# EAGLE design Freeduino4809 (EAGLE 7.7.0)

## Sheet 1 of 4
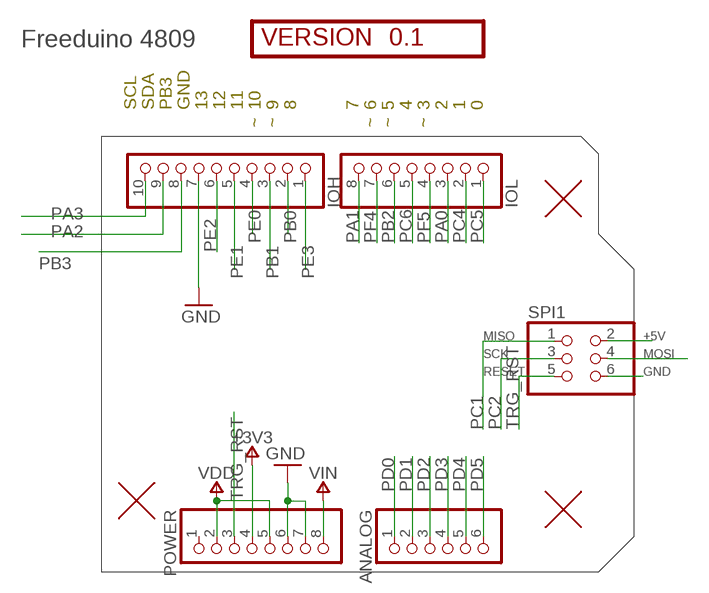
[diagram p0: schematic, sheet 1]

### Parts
ANALOG  Analog  PINHD-1X06TH  [1X06-TH]
IOH  Digital  PINHD-1X10TH  [1X10]
IOL  Digital  PINHD-1X08-DIGITALTH  [1X08]
POWER  Power  PINHD-1X08-POWERTH  [1X08]
SPI1  -  PINHD-2X03-ICSPTH  [2X03]
U$1  FIDUCIAL1.5X3  [FIDUCIAL-1.5X3]
U$2  FIDUCIAL1.5X3  [FIDUCIAL-1.5X3]
U$3  FIDUCIAL1.5X3  [FIDUCIAL-1.5X3]
VERSION  0.1  VERSION  [VERSION-NUMBER]

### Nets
+3V3: POWER.4 ; also sheet 4
GND: IOH.7 POWER.6 POWER.7 SPI1.6 ; also sheet 2,3,4
PA0: IOL.3 ; also sheet 2
PA1: IOL.8 ; also sheet 2
PA2: IOH.9 ; also sheet 2
PA3: IOH.10 ; also sheet 2
PB0: IOH.2 ; also sheet 2
PB1: IOH.3 ; also sheet 2
PB2: IOL.6 ; also sheet 2
PB3: IOH.8 ; also sheet 2
PC0: SPI1.4 ; also sheet 2
PC1: SPI1.1 ; also sheet 2
PC2: SPI1.3 ; also sheet 2
PC4: IOL.2 ; also sheet 2
PC5: IOL.1 ; also sheet 2
PC6: IOL.5 ; also sheet 2
PD0: ANALOG.1 ; also sheet 2
PD1: ANALOG.2 ; also sheet 2
PD2: ANALOG.3 ; also sheet 2
PD3: ANALOG.4 ; also sheet 2
PD4: ANALOG.5 ; also sheet 2
PD5: ANALOG.6 ; also sheet 2
PE0: IOH.4 ; also sheet 2
PE1: IOH.5 ; also sheet 2
PE2: IOH.6 ; also sheet 2
PE3: IOH.1 ; also sheet 2
PF4: IOL.7 ; also sheet 2
PF5: IOL.4 ; also sheet 2
TRG_RST: POWER.3 SPI1.5 ; also sheet 2,3
VDD [power]: POWER.2 POWER.5 SPI1.2 ; also sheet 2,3,4
VIN_EXT [power]: POWER.8 ; supply symbol labelled VIN ; also sheet 4
Unconnected: POWER.1

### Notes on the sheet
- Freeduino 4809
- SCL | SDA | PB3 | GND | 13 | 12 | 11 | 10 | 9 | 8 | 7 | 6 | 5 | 4 | 3 | 2 | 1 | 0
- ~ | ~ | ~ | ~ | ~

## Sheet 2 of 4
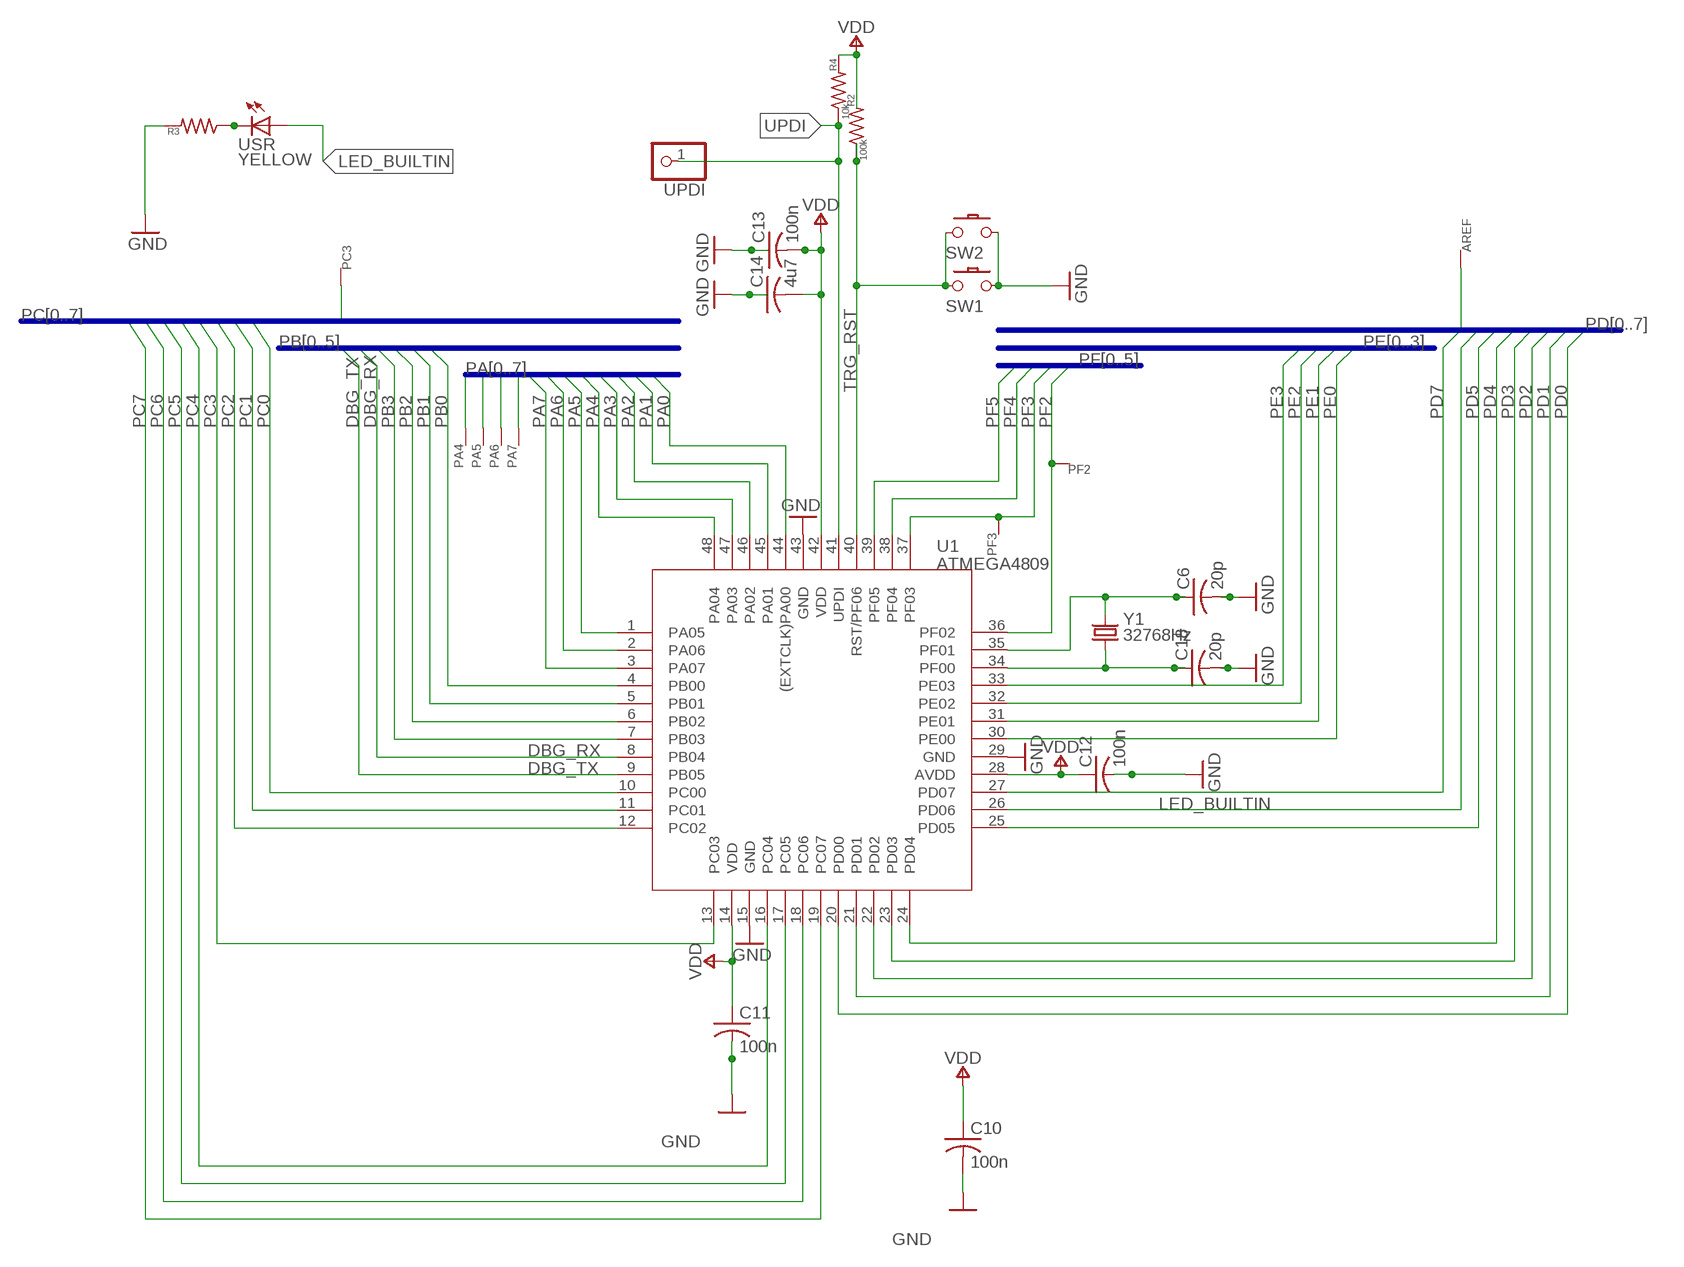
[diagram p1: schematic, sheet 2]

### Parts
AREF  WIRE-R10  [VIA10]
C6  20p  C-USC0805  [C0805]
C10  100n  C-USC0805  [C0805]
C11  100n  C-USC0805  [C0805]
C12  100n  C-USC0805  [C0805]
C13  100n  C-USC0805  [C0805]
C14  4u7  C-USC0805  [C0805]
C18  20p  C-USC0805  [C0805]
PA4  WIRE-R6  [VIA6]
PA5  WIRE-R6  [VIA6]
PA6  WIRE-R6  [VIA6]
PA7  WIRE-R6  [VIA6]
PC3  WIRE-R6  [VIA6]
PF2  WIRE-R6  [VIA6]
PF3  WIRE-R6  [VIA6]
R2  100k  R-US_R0805  [R0805]
R3  R-US_R0805  [R0805]
R4  10k  R-US_R0805  [R0805]
SW1  SW-PB2-NS/4MM  [SW-PB-SMT4MM]
SW2  SW-PB2-NSS52MM\  [SW-PB-SMT52MM]
U1  ATMEGA4809  [TQFP48]
UPDI  PINHD-1X1  [1X01]
USR  YELLOW  LED-YELLOW-0805  [CHIPLED_0805]
Y1  32768Hz  32.768KHZ  [ABS07]

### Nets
DBG_RX: U1.8(PB04) ; also sheet 3
DBG_TX: U1.9(PB05) ; also sheet 3
GND: C6.2 C10.2 C11.2 C12.2 C13.1 C14.1 C18.2 R3.2 SW1.P$4 SW2.S1 U1.15(GND) U1.29(GND) U1.43(GND) ; also sheet 1,3,4
LED_BUILTIN: U1.26(PD06) USR.A
N$4: C18.1 U1.34(PF00) Y1.1
N$5: C6.1 U1.35(PF01) Y1.2
N$22: R3.1 USR.C
PA0: U1.44((EXTCLK)PA00) ; also sheet 1
PA1: U1.45(PA01) ; also sheet 1
PA2: U1.46(PA02) ; also sheet 1
PA3: U1.47(PA03) ; also sheet 1
PA4: PA4.P$1 U1.48(PA04)
PA5: PA5.P$1 U1.1(PA05)
PA6: PA6.P$1 U1.2(PA06)
PA7: PA7.P$1 U1.3(PA07)
PB0: U1.4(PB00) ; also sheet 1
PB1: U1.5(PB01) ; also sheet 1
PB2: U1.6(PB02) ; also sheet 1
PB3: U1.7(PB03) ; also sheet 1
PC0: U1.10(PC00) ; also sheet 1
PC1: U1.11(PC01) ; also sheet 1
PC2: U1.12(PC02) ; also sheet 1
PC3: PC3.P$1 U1.13(PC03)
PC4: U1.16(PC04) ; also sheet 1
PC5: U1.17(PC05) ; also sheet 1
PC6: U1.18(PC06) ; also sheet 1
PC7: U1.19(PC07)
PD0: U1.20(PD00) ; also sheet 1
PD1: U1.21(PD01) ; also sheet 1
PD2: U1.22(PD02) ; also sheet 1
PD3: U1.23(PD03) ; also sheet 1
PD4: U1.24(PD04) ; also sheet 1
PD5: U1.25(PD05) ; also sheet 1
PD7: AREF.P$1 U1.27(PD07)
PE0: U1.30(PE00) ; also sheet 1
PE1: U1.31(PE01) ; also sheet 1
PE2: U1.32(PE02) ; also sheet 1
PE3: U1.33(PE03) ; also sheet 1
PF2: PF2.P$1 U1.36(PF02)
PF3: PF3.P$1 U1.37(PF03)
PF4: U1.38(PF04) ; also sheet 1
PF5: U1.39(PF05) ; also sheet 1
TRG_RST: R2.1 SW1.P$2 SW2.C2 U1.40(RST/PF06) ; also sheet 1,3
UPDI: R4.1 U1.41(UPDI) UPDI.1
VDD [power]: C10.1 C11.1 C12.1 C13.2 C14.2 R2.2 R4.2 U1.14(VDD) U1.28(AVDD) U1.42(VDD) ; also sheet 1,3,4

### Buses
PA[0..7]
PB[0..5]
PF[0..5]
PE[0..3]
PD[0..7]
PC[0..7]

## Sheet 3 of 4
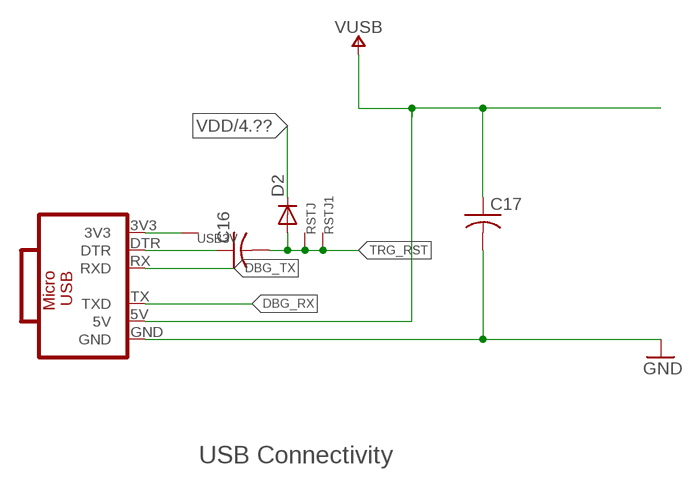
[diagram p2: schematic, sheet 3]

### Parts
C16  C-USC0805  [C0805]
C17  C-USC0805  [C0805]
D2  DIODE-SIGNAL-SOD323  [SOD323F]
RSTJ  WIRE-VIA8  [VIA8]
RSTJ1  WIRE-VIA8  [VIA8]
USB3V  WIRE-VIA8  [VIA8]
USBMOD  CH340E-MODNOHOLES  [CH340E-MOD-NOHOLES]

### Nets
DBG_RX: USBMOD.TX(TXD) ; also sheet 2
DBG_TX: USBMOD.RX(RXD) ; also sheet 2
DTR: C16.1 USBMOD.DTR
GND: C17.2 USBMOD.GND ; also sheet 1,2,4
TRG_RST: C16.2 D2.A RSTJ1.P$1 RSTJ.P$1 ; also sheet 1,2
USB3V: USB3V.P$1 USBMOD.3V3
VDD [power]: D2.C ; also sheet 1,2,4
VUSB: C17.1 USBMOD.5V ; also sheet 4

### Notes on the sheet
- USB Connectivity

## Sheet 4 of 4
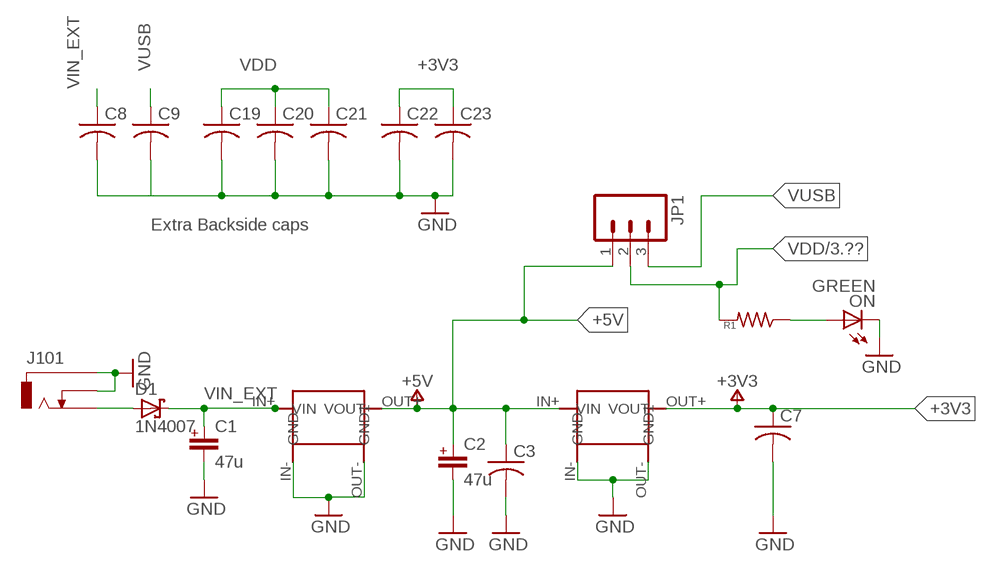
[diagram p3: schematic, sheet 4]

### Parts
C1  47u  C+-47UFPAN-D  [PANASONIC_D]
C2  47u  C+-47UFPAN-D  [PANASONIC_D]
C3  C-USC0805  [C0805]
C7  C-USC0805  [C0805]
C8  C-USC0805  [C0805]
C9  C-USC0805  [C0805]
C19  C-USC1206  [C1206]
C20  C-USC1206  [C1206]
C21  C-USC0805  [C0805]
C22  C-USC1206  [C1206]
C23  C-USC0805  [C0805]
D1  1N4007  D_SCHOTTKY-4007-SMB  [SMB_DO214AA]
J101  -  BARRELLG  [POWERSUPPLY_DC-21MM]
JP1  M03LOCK_LONGPADS  [1X03_LOCK_LONGPADS]
ON  GREEN  LED-GREEN-0805  [CHIPLED_0805]
R1  R-US_R0805  [R0805]
VREG-3V3  VREG-4-MOD  [VREG-4-11X17]
VREG-5V  VREG-4-MOD  [VREG-4-11X17]

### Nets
+3V3: C7.1 C22.1 C23.1 VREG-3V3.OUT+(VOUT) ; also sheet 1
+5V: C2.+ C3.1 JP1.1 VREG-3V3.IN+(VIN) VREG-5V.OUT+(VOUT)
GND: C1.- C2.- C3.2 C7.2 C8.2 C9.2 C19.2 C20.2 C21.2 C22.2 C23.2 J101.-1 J101.-2 J101.-3 J101.E1 J101.E2 J101.E3 ON.C VREG-3V3.IN-(GND) VREG-3V3.OUT-(GND1) VREG-5V.IN-(GND) VREG-5V.OUT-(GND1) ; also sheet 1,2,3
N$1: D1.A J101.+1 J101.+2 J101.+3
N$2: ON.A R1.1
VDD [power]: C19.1 C20.1 C21.1 JP1.2 R1.2 ; also sheet 1,2,3
VIN_EXT [power]: C1.+ C8.1 D1.C VREG-5V.IN+(VIN) ; also sheet 1
VUSB: C9.1 JP1.3 ; also sheet 3

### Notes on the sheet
- Extra Backside caps

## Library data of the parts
ANALOG = Arduino-connectors:PINHD-1X06: PIN HEADER; CODE-ARDUINO: 3649; DATASHEET: -; DISTRIBUTOR-LINK: -; DISTRIBUTOR-PN: -; MANUFACTURER: -; MANUFACTURER-PN: FH254-106DF085149V
AREF PA4-PA7 PC3 PF2 PF3 RSTJ RSTJ1 USB3V = mylib4:WIRE: Pad for a wire offboard
C1 C2 = Arduino-rcl:C+: Polarized Capacitor; CODE-ARDUINO: 0113; DATASHEET: https://industrial.panasonic.com/cdbs/www-data/pdf/RDE0000/DME0000COL90.pdf; DISTRIBUTOR-LINK: https://www.digikey.com/product-detail/en/panasonic-electronic-components/EEE-1EA470WP/PCE3908CT-ND/766284; DISTRIBUTOR-PN: PCE3908CT-ND; MANUFACTURER: Panasonic; MANUFACTURER-PN: EEE-1EA470WP; PN-ALTERNATIVE1: TS13C01E470MET000R
C3 C6-C14 C16-C23 = my-rcl:C-US: CAPACITOR, American symbol
D1 = Arduino-diodes:D_SCHOTTKY: Schottky Diodes; CODE-ARDUINO: 0020; DATASHEET: www.comchiptech.com/cms/UserFiles/CGRA4001-G%20Thru.%20CGRA4007-HF%20RevD.pdf; DISTRIBUTOR-LINK: https://www.digikey.com/product-detail/en/comchip-technology/CGRA4007-G/641-1018-1-ND/1121140; DISTRIBUTOR-PN: 641-1018-1-ND; MANUFACTURER: Comchip; MANUFACTURER-PN: CGRA4007-G; PN-ALTERNATIVE1: 1N4007SMA
D2 = mylib4:DIODE-SIGNAL
IOH = Arduino-connectors:PINHD-1X10: PIN HEADER; CODE-ARDUINO: 3648; DATASHEET: -; DISTRIBUTOR-LINK: -; DISTRIBUTOR-PN: -; MANUFACTURER: -; MANUFACTURER-PN: FH254-110DF085149V
IOL = Arduino-connectors:PINHD-1X08: PIN HEADER; CODE-ARDUINO: 3648; DATASHEET: -; DISTRIBUTOR-LINK: -; DISTRIBUTOR-PN: -; MANUFACTURER: -; MANUFACTURER-PN: FH254-108DF085149V
J101 = Arduino-connectors:BARREL: Power Barrel Connector Jack 2.10mm ID (0.083"), 5.50mm OD (0.217") Through Hole, Right Angle; CODE-ARDUINO: 0018; DATASHEET: http://www.mouser.com/ds/2/253/KC-301287-195995.pdf; DISTRIBUTOR-LINK: https://www.mouser.it/ProductDetail/Kobiconn/163-179PH-EX/?qs=Xb8IjHhkxj5l2UOaIqcGCw==; DISTRIBUTOR-PN: 163-179PH-EX; MANUFACTURER: Kobiconn; MANUFACTURER-PN: 163-179PH-EX
JP1 = SparkFun:M03: Header 3 Standard 3-pin 0.1" header. Use with straight break away headers (SKU : PRT-00116), right angle break away headers (PRT-00553), swiss pins (PRT-00743), machine pins (PRT-00117), and female headers (PRT-00115). Molex polarized connector foot print use with SKU : PRT-08232 with associated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
ON = Arduino-diodes:LED: LED; CODE-ARDUINO: 0043; DATASHEET: https://media.digikey.com/pdf/Data%20Sheets/Lite-On%20PDFs/LTST-C170GKT.pdf; DISTRIBUTOR-LINK: https://www.digikey.com/product-detail/it/lite-on-inc/LTST-C170GKT/160-1179-1-ND/269251; DISTRIBUTOR-PN: 160-1179-1-ND; MANUFACTURER: Lite-On; MANUFACTURER-PN: LTST-C170GKT; PN-ALTERNATIVE1: KPT-2012SGC
POWER = Arduino-connectors:PINHD-1X08: PIN HEADER; CODE-ARDUINO: 3649; DATASHEET: -; DISTRIBUTOR-LINK: -; DISTRIBUTOR-PN: -; MANUFACTURER: -; MANUFACTURER-PN: FH254-108DF085149V
R1-R4 = my-rcl:R-US_: RESISTOR, American symbol
SPI1 = Arduino-connectors:PINHD-2X03-ICSP: PIN HEADER; CODE-ARDUINO: 0114; DATASHEET: -; DISTRIBUTOR-LINK: https://www.digikey.com/product-detail/en/samtec-inc/TSW-103-25-S-D/TSW-103-25-S-D-ND/7863771; DISTRIBUTOR-PN: TSW-103-25-S-D-ND; MANUFACTURER: Samtec; MANUFACTURER-PN: TSW-103-25-S-D
SW1 SW2 = mylib4:SW-PB2-NS: SPST switch with no shield
U1 = Arduino-ucs&SoCs:ATMEGA4809: ATMEGA4809; CODE-ARDUINO: 2322; DATASHEET: http://ww1.microchip.com/downloads/en/DeviceDoc/40002016A.pdf; DISTRIBUTOR-LINK: https://www.digikey.com/product-detail/en/microchip-technology/ATMEGA4809-AFR/ATMEGA4809-AFRCT-ND/8540756; DISTRIBUTOR-PN: ATMEGA4809-AFRCT-ND; MANUFACTURER: Microchip; MANUFACTURER-PN: ATMEGA4809-AFR
U$1-U$3 = SparkFunEagle-6-6-07:FIDUCIAL: Fiducial Alignment Points
UPDI = pinhead:PINHD-1X1: PIN HEADER
USBMOD = mini-usb:CH340E-MOD
USR = Arduino-diodes:LED: LED; CODE-ARDUINO: 0044; DATASHEET: https://media.digikey.com/pdf/Data%20Sheets/Lite-On%20PDFs/LTST-C170GKT.pdf; DISTRIBUTOR-LINK: https://www.digikey.com/product-detail/it/lite-on-inc/LTST-C170YKT/160-1175-1-ND/269247; DISTRIBUTOR-PN: 160-1175-1-ND; MANUFACTURER: Lite-On; MANUFACTURER-PN: LTST-C170YKT; PN-ALTERNATIVE1: KPT-2012YC
VERSION = mylib4:VERSION: Version number for drawings
VREG-3V3 VREG-5V = mylib4:VREG-4-MOD
Y1 = Arduino-crystals:32.768KHZ: LF crystal; CODE-ARDUINO: 0213; DATASHEET: http://www.abracon.com/Resonators/ABS07.pdf; DISTRIBUTOR-LINK: http://www.digikey.com/product-detail/en/abracon-llc/ABS07-32.768KHZ-T/535-9542-1-ND/1237009; DISTRIBUTOR-PN: 535-9542-1-ND; MANUFACTURER: Abracon LLC; MANUFACTURER-PN: ABS07-32.768KHZ-T

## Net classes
0 default: width 0.2 mm, drill 0.5 mm
1 power: width 0.6 mm

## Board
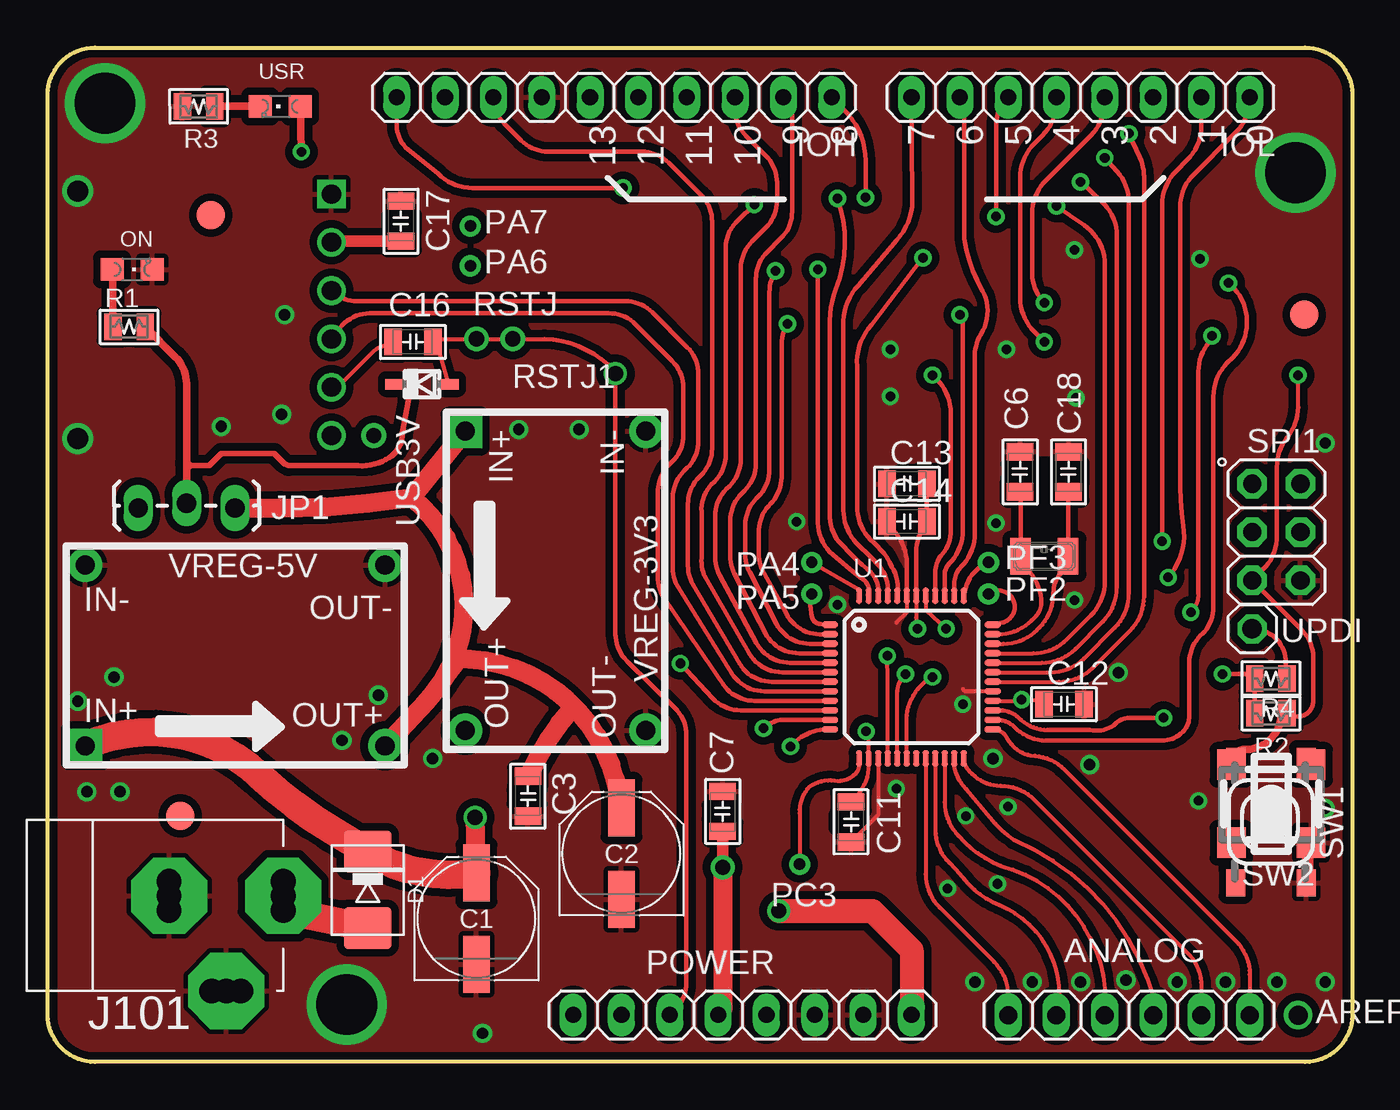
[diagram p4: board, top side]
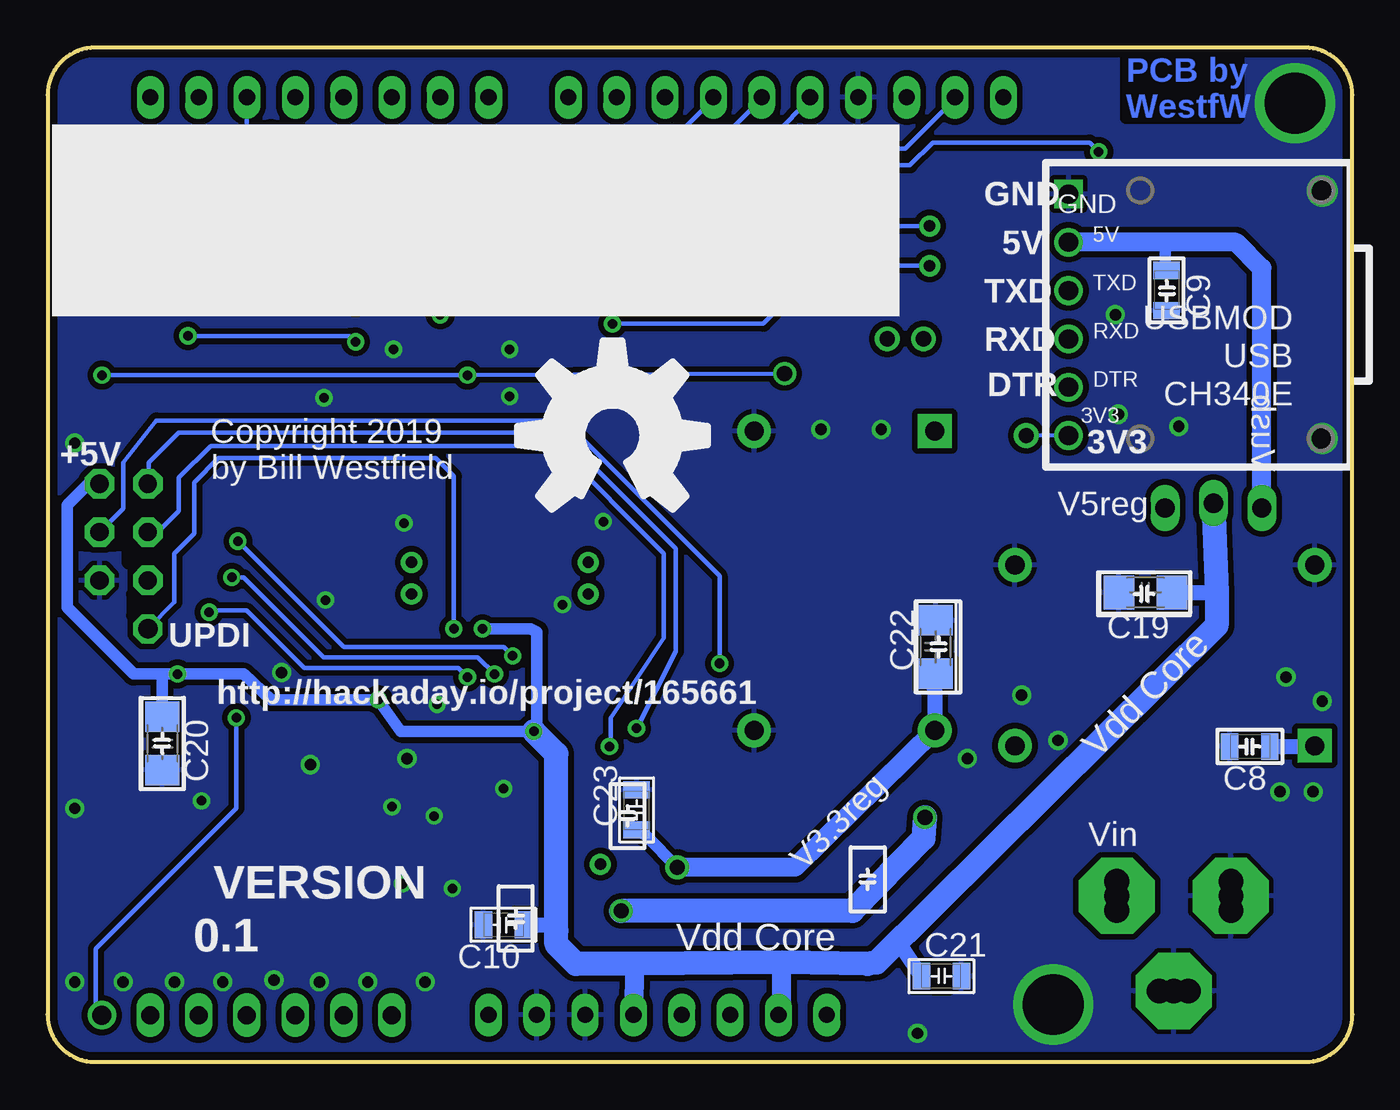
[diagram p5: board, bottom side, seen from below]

Size 68.58 x 53.34 mm. Coordinates in mm from the lower left corner, seen from the top.
Outline: 0,50.84 arc-90 2.5,53.34 66.08,53.34 arc-90 68.58,50.84 68.58,2.5 arc-90 66.08,0 2.5,0 arc-90 0,2.5 0,50.84
Copper layers (1*16): Top 0.035mm / dielectric 1.5mm / Bottom 0.035mm
Design rules "default *": minimum track width 8mil, minimum drill 0.3mm, track to track 6mil, track to pad 6mil, pad to pad 6mil, via to via 6mil, smd to smd 6mil, copper to edge 16mil, drill to drill 8mil, minimum pad ring 10mil, minimum via ring 8mil, stop-mask expansion 4mil, vias tented up to drill 0.55mm, thermal gap 10mil
tRestrict: area 52.1,25.6 to 52.8,30.5; area 50.5,30.7 to 51.8,31.4; area 53,30.8 to 54.4,31.5; area 51.8,30.7 to 53.1,31.4; area 44.8,29.7 to 45.5,31; area 44.8,27.8 to 45.6,29.1; area 18.8,37.2 to 19.5,38.6; area 17.9,43.8 to 19.3,44.5; area 34.8,12.8 to 36.1,13.5; area 41.4,12.3 to 42.8,13; area 24.5,13.6 to 25.9,14.3; area 3.9,38 to 4.6,39.3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
bRestrict: area 10.5,24 to 11.3,25.2; area 9,40.1 to 10.3,40.9; area 4.9,16 to 5.7,17.2; area 21.3,21.5 to 22.5,22.3; area 21.2,3.8 to 22,5.1; area 37.1,12.9 to 38.3,13.7; area 44.2,6.6 to 45,7.8; area 61.8,16.4 to 63.1,17.1; area 30.7,4.6 to 37.1,5.6; 6 lines

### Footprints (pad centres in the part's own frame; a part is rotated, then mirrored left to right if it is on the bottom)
1X06-TH = drill 0.95 pad 1.422 long: 1 -6.35,0; 2 -3.81,0; 3 -1.27,0; 4 1.27,0; 5 3.81,0; 6 6.35,0
VIA10 = drill 1: P$1 0,0
PANASONIC_D = smd 3 x 1.4: + 2.4,0; - -2.4,0
C0805 = smd 0.914 x 1.397: 1 -1.053,0; 2 1.053,0
C1206 = smd 1.6 x 1.8: 1 -1.4,0; 2 1.4,0
SMB_DO214AA = smd 2.2 x 2.5: A -2,0; C 2,0
SOD323F = smd 0.55 x 1.05: A 0,-1.4; C 0,1.4
1X10 = drill 0.85 pad 1.422 long: 1 -11.43,0; 2 -8.89,0; 3 -6.35,0; 4 -3.81,0; 5 -1.27,0; 6 1.27,0; 7 3.81,0; 8 6.35,0; 9 8.89,0; 10 11.43,0
1X08 = drill 0.85 pad 1.422 long: 1 -8.89,0; 2 -6.35,0; 3 -3.81,0; 4 -1.27,0; 5 1.27,0; 6 3.81,0; 7 6.35,0; 8 8.89,0
POWERSUPPLY_DC-21MM = drill 1.3 pad 4 octagon: +1 -0.076,-6.35; -1 -0.076,-0.356; E1 -5.08,-3.353 | drill 1.3: +2 -0.838,-6.35; +3 0.686,-6.35; -2 -0.838,-0.356; -3 0.686,-0.356; E2 -5.08,-2.591; E3 -5.08,-4.115
1X03_LOCK_LONGPADS = drill 1.016 long: 1 0,0; 2 2.54,-0.254; 3 5.08,0
CHIPLED_0805 = smd 1.2 x 1.2: A -1.05,0; C 1.05,0
VIA6 = drill 0.6: P$1 0,0
R0805 = smd 0.914 x 1.397: 1 -0.85,0; 2 0.85,0
VIA8 = drill 0.8: P$1 0,0
2X03 = drill 0.95 pad 1.55 octagon: 1 2.54,1.27; 2 2.54,-1.27; 3 0,1.27; 4 0,-1.27; 5 -2.54,1.27; 6 -2.54,-1.27
SW-PB-SMT4MM = smd 1.4 x 1: P$1 -3.2,1.85; P$2 -3.2,-1.85; P$3 3.2,-1.85; P$4 3.2,1.85
SW-PB-SMT52MM = smd 1.5 x 1.6: C1 2.1,2.05; C2 2.1,-2.05; S1 -2.1,2.05; S2 -2.1,-2.05
TQFP48 = smd 0.85 x 0.32: 1 -4.275,2.75; 2 -4.275,2.25; 3 -4.275,1.75; 4 -4.275,1.25; 5 -4.275,0.75; 6 -4.275,0.25; 7 -4.275,-0.25; 8 -4.275,-0.75; 9 -4.275,-1.25; 10 -4.275,-1.75; 11 -4.275,-2.25; 12 -4.275,-2.75; 25 4.275,-2.75; 26 4.275,-2.25; 27 4.275,-1.75; 28 4.275,-1.25; 29 4.275,-0.75; 30 4.275,-0.25; 31 4.275,0.25; 32 4.275,0.75; 33 4.275,1.25; 34 4.275,1.75; 35 4.275,2.25; 36 4.275,2.75 | smd 0.32 x 0.85: 13 -2.75,-4.275; 14 -2.25,-4.275; 15 -1.75,-4.275; 16 -1.25,-4.275; 17 -0.75,-4.275; 18 -0.25,-4.275; 19 0.25,-4.275; 20 0.75,-4.275; 21 1.25,-4.275; 22 1.75,-4.275; 23 2.25,-4.275; 24 2.75,-4.275; 37 2.75,4.275; 38 2.25,4.275; 39 1.75,4.275; 40 1.25,4.275; 41 0.75,4.275; 42 0.25,4.275; 43 -0.25,4.275; 44 -0.75,4.275; 45 -1.25,4.275; 46 -1.75,4.275; 47 -2.25,4.275; 48 -2.75,4.275 | smd 0 x 0: EP 0,0
FIDUCIAL-1.5X3 = smd 1.5 x 1.5: 1 0,0
1X01 = drill 1.016 octagon: 1 0,0
CH340E-MOD-NOHOLES = drill 1: 3V3 6.35,6.35; 5V 6.35,-3.81; DTR 6.35,3.81; RX 6.35,1.27; TX 6.35,-1.27 | drill 1 square: GND 6.35,-6.35
VREG-4-11X17 = drill 1 pad 1.778 square: IN+ -5,-2.5 | drill 1 pad 1.778: IN- -5,7; OUT+ 10.75,-2.5; OUT- 10.75,7
ABS07 = smd 1.1 x 1.9: 1 -1.25,0; 2 1.25,0

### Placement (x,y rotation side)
ANALOG  56.83,2.46 0 top
AREF  65.72,2.46 0 top
C1  22.54,7.54 90 top
C2  30.16,10.95 90 top
C3  25.24,13.97 270 top
C6  51.12,31.04 90 top
C7  35.48,13.18 90 top
C8  5.4,16.59 180 bottom
C9  9.76,40.56 270 bottom
C10  44.63,7.21 180 bottom
C11  42.23,12.62 270 top
C12  53.42,18.81 0 top
C13  45.16,30.4 0 top
C14  45.16,28.42 0 top
C16  19.21,37.86 0 top
C17  18.57,44.21 90 top
C18  53.66,31.04 90 top
C19  10.87,24.69 180 bottom
C20  62.55,16.75 270 bottom
C21  21.6,4.52 0 bottom
C22  21.91,21.83 90 bottom
C23  37.62,13.26 90 bottom
D1  16.83,9.05 90 top
D2  19.69,35.64 90 top
IOH  29.78,50.72 180 top
IOL  54.29,50.72 180 top
J101  6.03,8.81 90 top
JP1  9.84,29.13 180 top
ON  4.45,41.67 0 top
PA4  40.16,26.27 0 top
PA5  40.16,24.61 0 top
PA6  22.23,41.86 0 top
PA7  22.23,43.96 0 top
PC3  39.53,10.4 0 top
PF2  49.45,24.61 0 top
PF3  49.45,26.27 0 top
POWER  36.51,2.47 0 top
R1  4.29,38.66 0 top
R2  64.29,18.34 180 top
R3  7.94,50.24 180 top
R4  64.29,20.16 180 top
RSTJ  22.54,38.02 0 top
RSTJ1  24.45,38.02 0 top
SPI1  64.58,27.86 90 top
SW1  64.29,12.62 270 top
SW2  64.31,13.58 180 top
U1  45.4,20.24 0 top
U$1  6.99,12.94 0 top
U$2  66.04,39.29 0 top
U$3  8.57,44.53 0 top
UPDI  63.31,22.78 0 top
USB3V  17.14,32.94 0 top
USBMOD  8.57,39.29 180 bottom
USR  12.22,50.24 180 top
VERSION  not placed on the board
VREG-3V3  24.45,28.18 270 top
VREG-5V  6.99,19.13 0 top
Y1  52.39,26.59 180 top

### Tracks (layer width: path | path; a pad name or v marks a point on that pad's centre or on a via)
+3V3  (via drill 0.8 pad 1.27)
  Top 0.6: C7.1 v35.48,10.24
  Top 1: v35.48,10.24 35.48,2.71 POWER.4
  Bottom 0.6: C22.1 arc-90 21.95,19.46 | C23.1 37.13,11.88 v35.48,10.24
  Bottom 0.8: 21.95,19.46 VREG-3V3.OUT+
  Bottom 1: VREG-3V3.OUT+ 29.29,10.24 v35.48,10.24
+5V
  Top 0.6: 29.85,14.84 28.34,17.86 27.54,18.57 | 30.24,13.33 C2.+
  Top 1: C2.+ 30.24,13.35 | JP1.1 12.22,29.13 arc9 19.13,29.69 | VREG-5V.OUT+ 19.92,18.97 | 19.92,18.97 arc95 19.13,29.69 | 19.13,29.69 VREG-3V3.IN+ | 30.24,13.33 29.85,14.84 arc77 21.35,21.19 21.35,20.88 19.92,18.97 | C3.1 25.4,15.24 arc-17 27.54,18.57
DBG_RX
  Top 0.229: U1.8 37.66,19.49 arc-58 35.96,20.43 33.16,24.91 arc-32 32.86,25.97 32.86,29.65 arc-45 33.45,31.07 33.62,31.24 arc45 34.21,32.66 34.21,36.16 arc45 33.62,37.57 31.78,39.42 arc45 30.37,40 16.26,40 arc-45 USBMOD.TX
DBG_TX
  Top 0.229: U1.9 37.15,18.99 arc-56 35.5,19.86 32.5,24.25 arc-34 32.07,25.38 32.07,30.05 arc-45 32.73,31.46 32.83,31.56 arc45 33.42,32.98 33.42,35.45 arc45 32.83,36.86 30.91,38.78 arc45 29.49,39.37 16.94,39.37 arc53 15.35,38.58 USBMOD.RX
DTR
  Top 0.203: USBMOD.DTR 15.24,35.48 17.08,37.33 arc-45 18,37.7 C16.1
GND  (via drill 0.5, 0.6, 1.1, 3.2)
  Top 0.203: U1.15 43.65,12.99 C11.2 | U1.29 48.22,19.49 48.1,19.61 | U1.43 45.15,23.64 44.61,23.1
  Top 0.229: U1.43 45.15,26.24 arc45 44.45,27.94 arc45 44.35,28.17 C14.1
  Top 0.6: SW2.S1 arc90 66.22,11.33 66.22,9.29
  other vias: 54.29,4.21 56.68,4.31 59.37,4.21 61.91,4.21 47.31,9.13 49.69,15.95 50.48,13.41 48.26,12.94 51.75,4.21 49.93,9.37 54.77,15.64 56.28,20.48 64.61,4.21 48.74,4.21 41.51,24.05 48.1,18.81 44.61,14.37 44.29,37.47 44.29,35 54.05,34.93 50.4,37.47 53.97,42.7 60.56,42.23 39.37,28.42 49.85,28.34 53.97,24.29 1.59,45.8 1.59,32.78 67.15,4.21 67.15,13.34 67.15,32.54 1.59,18.97 3.49,20.24 3.81,14.21 2.06,14.21 22.86,1.51 24.77,33.26 27.94,33.26 20.24,15.95 60.48,13.73 9.13,33.42 12.3,34.05 12.46,39.29 17.38,19.29 15.48,16.91 3.02,50.42 65.58,46.77 15.72,3.02
  pour Top (isolate 0.4): -2.86,55.8 72.71,55.8 72.71,-3.25 -2.86,-3.25
  pour Bottom (isolate 0.3): -0.64,55.17 70.17,55.17 70.17,-1.98 -0.64,-1.98 -0.64,53.26
LED_BUILTIN  (via drill 0.5)
  Top 0.203: U1.26 49.93,17.99 arc-45 50.78,17.64 arc45 52.47,16.91
  Top 0.229: v62.07,40.96 62.21,40.83 arc-47 63.02,38.98 63.02,38.82 arc-45 62.29,37.05 62.01,36.77 arc45 61.28,35 61.28,23.93 arc-45 60.69,22.51 60.59,22.41 arc45 60.01,21 60.01,18.19 arc-45 59.66,17.36 arc-45 58.58,16.91 52.47,16.91
  Top 0.4: USR.A v13.33,47.86
  Bottom 0.229: v62.07,40.96 62.07,41.04 54.93,41.04 54.45,41.51 47.7,41.51 46.67,40.48 42.78,40.48 40,43.74 34.45,43.74 31.09,47.09 arc45 30.96,47.15 23.26,47.15 22.07,48.34 13.81,48.34 v13.33,47.86
N$1
  Top 1.5: J101.+2 D1.A
  Bottom 0.2: J101.+2 J101.+1 | J101.+3 J101.+1 | 12.38,7.94 J101.+1
N$2
  Top 0.4: ON.A 3.44,40.84 R1.1
N$4
  Top 0.203: U1.34 50.24,21.99 arc45 52.01,22.72 52.13,22.84 arc45 52.86,24.61 52.86,24.65
  Top 0.229: C18.1 53.64,29.96 Y1.1 53.34,26.29 53.34,25.8 arc45 52.86,24.65
N$5
  Top 0.203: U1.35 49.95,22.49 arc45 51.72,23.22 51.95,23.45 arc45 52.23,24.13
  Top 0.229: C6.1 51.14,29.96 Y1.2 51.43,26.29 51.43,25.96 51.5,25.89 arc-45 52.23,24.13
N$22
  Top 0.4: R3.1 USR.C
PA0  (via drill 0.5)
  Top 0.229: v46.01,42.28 43.31,38.78 arc46 42.54,36.58 42.54,29.23 arc49 43.42,27.3 arc-26 44.37,26.03 arc-40 U1.44
  Bottom 0.229: IOL.3 58.1,48.34 53.18,43.42 46.99,43.42 v46.01,42.28
PA1
  Top 0.229: IOL.8 45.45,45.54 arc-46 44.63,43.22 42.6,40.83 arc46 41.83,38.72 41.83,29.01 arc43 42.51,27.3 42.74,27.05 arc-2 43.64,26.17 arc-49 U1.45
PA2  (via drill 0.5)
  Top 0.229: U1.46 arc62 43.06,25.94 arc-7 42.34,26.57 41.57,27.37 arc-44 41.12,29.02 41.12,38.97 arc-22 41.43,40.64 arc41 v41.51,45.4
  Bottom 0.229: 41.47,45.44 v41.51,45.4 40.56,46.35 33.26,46.35 31.59,48.02 23.49,48.02 20.96,50.56 20.96,50.72 IOH.9
PA3  (via drill 0.5)
  Top 0.203: U1.47 arc-90 43.1,24.57 43.18,24.84
  Top 0.229: v40.48,41.67 40.48,28.55 arc44 41.1,26.82 arc2 42.7,25.48 arc-53 43.18,24.84 | v30.24,45.96 22.32,45.96 arc-45 20.53,46.7 18.81,48.1 arc-45 18.35,49.38 IOH.10
  Bottom 0.229: v40.48,41.67 40.32,41.91 39.45,42.78 33.42,42.78 v30.24,45.96
PA4
  Top 0.203: U1.48 42.62,24.84
  Top 0.229: 42.62,24.84 PA4.P$1
PA5
  Top 0.229: U1.1 40.64,23.02 arc-73 40.16,23.42 arc-27 PA5.P$1
PA6  (via drill 0.5)
  Top 0.229: U1.2 40.6,22.49 arc-63 38.81,23.58 38.66,23.89 37.54,25.91 arc-28 37.39,26.93 37.39,27.83 arc-45 37.89,29.24 37.99,29.34 arc45 38.58,30.75 38.58,37.73 arc-30 38.84,38.72 v38.89,38.81
  Bottom 0.229: v38.89,38.81 30.96,38.81 27.91,41.86 PA6.P$1
PA7  (via drill 0.5)
  Top 0.229: U1.3 40.07,21.99 arc-63 38.29,23.07 36.9,25.76 arc-27 36.67,26.68 36.67,28.22 arc-45 37.26,29.64 37.36,29.74 arc45 37.94,31.15 37.94,40.49 arc-27 38.15,41.38 v38.26,41.59
  Bottom 0.229: v38.26,41.59 30.8,41.59 28.43,43.96 PA7.P$1
PB0
  Top 0.229: U1.4 39.49,21.49 arc-63 37.72,22.57 36.1,25.68 arc-27 35.88,26.6 35.88,28.46 arc-45 36.46,29.88 36.64,30.05 arc45 37.23,31.47 37.23,41.16 arc-45 37.81,42.58 38.55,43.31 arc45 39.13,44.72 39.13,49.61 arc45 IOH.2
PB1
  Top 0.229: U1.5 39.02,20.99 arc-61 37.26,22.04 35.33,25.59 arc-29 35.08,26.54 35.08,28.7 arc-45 35.67,30.11 35.85,30.29 arc45 36.43,31.71 36.43,41.72 arc-45 37.02,43.13 37.75,43.86 arc45 38.34,45.28 38.34,46.24 arc45 37.75,47.66 36.7,48.71 arc-45 36.12,50.12 36.12,50.7 IOH.3
PB2  (via drill 0.5)
  Top 0.229: v49.85,44.45 49.85,49.19 arc-45 IOL.6 | U1.6 38.61,20.49 arc-60 36.88,21.49 34.56,25.49 arc-30 34.37,26.49 34.37,28.94 arc-45 34.88,30.35 35.05,30.53 arc45 35.64,31.94 35.64,42.8 arc-47 36.26,44.25 v37.15,45.08
  Bottom 0.229: v37.15,45.08 40,45.08 40.96,44.13 45.4,44.13 45.72,44.45 v49.85,44.45
PB3
  Top 0.229: U1.7 38.07,19.99 arc-60 36.34,20.98 33.93,25.09 arc-30 33.65,26.1 33.65,29.33 arc-45 34.24,30.75 34.34,30.85 arc45 34.92,32.26 34.92,44.18 arc45 34.34,45.59 32.65,47.28 arc45 31.24,47.86 26.31,47.86 arc-45 24.89,48.45 24,49.34 arc-45 IOH.8
PC0  (via drill 0.5)
  Top 0.229: U1.10 36.43,18.49 arc-47 34.97,19.12 v33.26,20.95
  Bottom 0.229: v33.26,20.95 33.26,25.56 41.43,33.73 62.86,33.73 64.61,31.51 64.61,29.1 SPI1.4
PC1  (via drill 0.5)
  Top 0.229: v37.62,17.54 arc-29 38.28,17.93 arc-16 38.71,17.99 U1.11
  Bottom 0.229: SPI1.1 63.26,30.45 63.26,31.51 61.67,33.1 41.67,33.1 35.56,26.99 35.56,21.59 v37.62,17.54
PC2  (via drill 0.5)
  Top 0.203: 40.99,17.49 U1.12
  Top 0.229: v39.05,16.59 39.22,16.76 arc-20 39.91,17.25 | 39.91,17.25 arc-25 40.99,17.49 | 39.93,17.22 39.91,17.25
  Bottom 0.229: 62.86,27.86 SPI1.3 62.79,27.86 61.67,28.97 61.67,30.72 60.01,32.38 41.83,32.38 36.2,26.75 36.2,22.3 38.97,18.1 38.97,16.67 v39.05,16.59
PC3
  Top 0.203: U1.13 42.65,15.65 arc-45 42.44,15.13 arc-45 41.55,14.76 arc45 40.02,14.46 arc45 39.53,13.09 PC3.P$1
PC4  (via drill 0.5)
  Top 0.203: U1.16 44.15,20.06 v44.13,21.35
  Top 0.229: IOL.2 60.64,49.22 arc-45 59.91,47.45 59.31,46.85 arc45 58.58,45.08 v58.58,27.38
  Bottom 0.229: v44.13,21.35 44.61,21.83 53.02,21.83 v58.58,27.38
PC5  (via drill 0.5)
  Top 0.203: U1.17 44.65,19.36 arc-45 v45.09,20.4
  Top 0.229: IOL.1 63.18,50.64 arc-45 62.45,48.88 60.1,46.53 arc45 59.53,44.68 59.53,30.24 arc9 59.69,28.18 arc-50 v58.9,25.48
  Bottom 0.229: v45.09,20.4 45.96,21.27 54.05,21.27 58.26,25.48 v58.9,25.48
PC6  (via drill 0.5)
  Top 0.203: 60.48,24.61 arc-45 v60.09,23.65 | U1.18 45.15,18 arc-45 45.88,19.77 46.35,20.24 v46.51,20.24
  Top 0.229: 60.48,24.61 60.48,36.3 arc-45 61.2,38.02 v61.2,38.18 | v52.39,37.86 51.85,38.4 arc-45 51.12,40.17 51.12,46.51 arc-45 51.85,48.28 52.29,48.72 arc45 53.02,50.49 IOL.5
  Bottom 0.229: v61.2,38.18 52.71,38.18 v52.39,37.86 | v46.51,20.24 46.99,20.72 55.09,20.72 58.1,23.73 60.01,23.73 v60.09,23.65
PD0
  Top 0.203: U1.20 46.15,9.89 arc45 46.88,8.12 49.75,5.26 arc-45 50.48,3.49 ANALOG.1
PD1
  Top 0.203: U1.21 46.67,15.95 46.67,12.23 arc45 47.4,10.46 arc-6 48.18,9.6 arc28 50.01,8.25 arc-54 53.02,4.76 arc-28 ANALOG.2
PD2
  Top 0.203: U1.22 47.15,13.65 arc45 47.88,11.88 arc27 50.09,10.32 arc-81 ANALOG.3
PD3
  Top 0.203: ANALOG.4 58.15,3.27 arc52 50.8,11.67 arc-17 49.53,12.86 48.29,14.34 arc-45 47.63,15.94 U1.23
PD4
  Top 0.203: U1.24 arc45 48.42,15.32 48.6,15.14 arc45 50.08,14.53 arc-45 51.85,13.79 59.91,5.73 arc-45 60.64,3.96 ANALOG.5
PD5
  Top 0.203: U1.25 arc-58 50.38,17.1 50.55,16.83 arc45 51.67,16.11 arc-45 53.44,15.38 62.45,6.37 arc-45 63.18,4.6 ANALOG.6
PD7  (via drill 0.5)
  Top 0.203: U1.27 50.07,18.49 arc-45 51.02,18.12 arc45 52.55,17.46
  Top 0.229: 52.55,17.46 54.79,17.46 arc45 56.04,17.7 arc-45 56.84,18.1 v58.66,18.1
  Bottom 0.229: v58.66,18.1 58.66,13.33 66.04,5.95 66.04,2.78 AREF.P$1 65.56,2.46
PE0  (via drill 0.5)
  Top 0.203: U1.30 53.17,19.99 arc45 54.93,20.72 56.89,22.68 arc45 57.63,24.45
  Top 0.229: 57.63,24.45 57.63,46.53 arc24 57.4,47.56 v56.83,48.82
  Bottom 0.229: IOH.4 33.65,50.72 33.65,50.56 35.72,48.5 54.05,48.5 54.37,48.82 v56.83,48.82
PE1  (via drill 0.5)
  Top 0.203: U1.31 52.71,20.49 arc45 54.48,21.22 56.1,22.84 arc45 56.83,24.61
  Top 0.229: 56.83,24.61 56.83,45.17 arc42 56.2,46.83 v55.56,47.55
  Bottom 0.229: v55.56,47.55 44.48,47.55 44.25,47.78 33.89,47.78 31.12,50.56 31.12,50.72 IOH.5
PE2  (via drill 0.5)
  Top 0.203: U1.32 52.26,20.99 arc45 54.03,21.72 55.47,23.16 arc45 56.2,24.93
  Top 0.229: 56.2,24.93 56.2,43.43 arc47 55.39,45.27 v54.29,46.28
  Bottom 0.229: 28.57,50.72 IOH.6 28.5,50.64 30.4,48.74 31.91,48.74 33.58,47.07 43.84,47.07 44.16,46.75 53.82,46.75 v54.29,46.28
PE3  (via drill 0.5)
  Top 0.203: U1.33 51.81,21.49 arc45 53.58,22.22 54.83,23.48
  Top 0.229: 54.83,23.48 arc45 55.56,25.24 55.56,41.94 arc55 54.48,44 v53.02,45.01 | v42.99,45.45 42.99,47.4 arc45 41.88,50.06 IOH.1
  Bottom 0.229: v53.02,45.01 51.91,45.88 43.51,45.88 v42.99,45.45
PF2
  Top 0.229: U1.36 50.17,23.1 arc206 PF2.P$1
PF3
  Top 0.229: U1.37 48.26,24.92 arc-53 PF3.P$1
PF4
  Top 0.229: U1.38 47.65,25.17 arc-45 48,26.02 arc45 48.74,27.78 48.74,37.15 arc-32 49.05,38.26 arc60 49.13,40.56 arc-22 48.18,43.28 48.18,50.64 IOL.7
PF5  (via drill 0.5)
  Top 0.229: U1.39 47.15,25.65 arc-45 47.37,26.18 arc45 48.1,27.94 48.1,39.13 v47.94,39.29 | v52.39,39.93 arc-45 51.75,41.46 51.75,44.6 arc-45 52.48,46.37 54.83,48.72 arc45 55.56,50.49 IOL.4
  Bottom 0.229: v47.94,39.29 48.58,39.93 v52.39,39.93
TRG_RST  (via drill 0.5, 0.8)
  Top 0.203: 65.72,34.43 v65.72,36.12 | 32.62,2.55 POWER.3 | D2.A 20.45,37.86 C16.2 20.26,38.02 RSTJ.P$1 RSTJ1.P$1 26.11,38.02
  Top 0.229: 65.72,34.43 arc-38 65.2,32.9 65.14,32.82 arc38 64.61,31.29 64.61,27.66 arc-45 63.88,25.89 SPI1.5 65.93,22.7 arc-45 66.52,21.29 66.52,18.97 arc-90 65.72,18.18 65.3,18.18 arc-90 R2.1 64.83,18.23 | 26.11,38.02 arc-45 29.78,36.34 v29.85,36.19 29.85,22.51 arc46 30.45,21.08 32.97,18.61 arc-46 33.58,17.18 33.58,4.18 arc-45 32.99,2.76 POWER.3 | U1.40 46.65,25.74 arc-45 47.05,26.73 arc45 47.47,28.1 47.47,34.13 arc45 46.73,35.9 v46.51,36.12 | SW1.P$2 62.36,15.82
  Top 0.4: 62.36,15.82 arc-90 62.86,16.43 arc90 64.83,18.23
  Top 0.6: SW2.C2 SW1.P$2
  Bottom 0.229: v65.72,36.12 v46.51,36.12 v29.85,36.19
UPDI  (via drill 0.5)
  Top 0.203: U1.41 46.15,23.78 v47.23,22.78
  Top 0.229: R4.1 arc-90 65.09,20.22 65.09,21 arc90 UPDI.1
  Bottom 0.203: 61.91,24.18 UPDI.1
  Bottom 0.229: 61.91,24.18 61.91,26.75 60.88,27.78 60.88,30.48 59.61,31.75 48.18,31.75 47.23,30.8 v47.23,22.78
USB3V
  Bottom 0.203: USBMOD.3V3 USB3V.P$1
VDD  (via drill 0.5)
  Top 0.203: C11.1 42.42,13.87 arc45 43.15,15.63 U1.14 43.15,17.2 v43.02,17.38 | U1.42 45.65,23.35 v45.72,22.78 | D2.C 18.64,35.61 arc-45 18.97,34.87 | U1.28 50.78,18.99 v51.2,19.05 52.13,19.05 C12.1 52.29,18.57
  Top 0.229: C13.2 C14.2 46.05,28.15 arc33 45.65,26.8 U1.42 | R2.2 R4.2 arc45 62.87,20.4 v61.75,20.4
  Top 0.3: 18.97,34.87 18.65,33.06 arc-53 17.97,31.77 arc-37 16.31,31.35 12.67,31.35 12.47,31.44 12.15,31.76 | 12.15,31.76 | 12.15,31.76 11.91,32 9.13,32 8.49,31.35 7.46,31.35
  Top 0.4: R1.2 6.72,37.08 arc-45 7.3,35.66 7.3,31.51 | 7.3,31.51 JP1.2 | 7.46,31.35 arc-90 7.3,31.51
  Bottom 0.6: v45.72,22.78 43.18,22.78 42.86,22.62 42.86,17.86 43.02,17.7 v43.02,17.38 50.01,17.38 v51.2,19.05 56.83,19.05 58.26,20.4 v61.75,20.4 62.55,20.4 | 62.55,20.4 64.06,20.4 67.55,23.89 67.55,29.29 66.44,30.4 SPI1.2 | C20.1 62.55,20.4
  Bottom 0.8: C19.1 7.14,24.69 | C21.1 23.81,6.25 25.48,5.16 | C10.1 42.15,7.21 41.84,6.91
  Bottom 1: POWER.2 30,2.47 30,5.24 | POWER.5 37.7,5.16
  Bottom 1.27: JP1.2 7.14,24.69 | 7.14,24.69 7.14,22.94 25,5.24 25.48,5.16 30,5.24 37.7,5.16 40.81,5.16 41.84,6.19 41.84,6.91 41.84,16.21 v43.02,17.38 | 7.14,24.69 arc-90 7.14,24.69
VIN_EXT  (via drill 0.8)
  Top 1: C1.+ arc90 C1.+ v22.47,12.86
  Top 1.27: v38.43,7.94 43.35,7.94 45.42,5.88 45.42,2.49 POWER.8
  Top 1.5: VREG-5V.IN+ arc-67 11.11,15.08 arc12 15,12.14 D1.C arc40 C1.+
  Bottom 0.6: 2.02,16.59 arc-90 VREG-5V.IN+
  Bottom 0.8: C8.1 2.02,16.59
  Bottom 1.27: v22.47,12.86 22.55,11.75 26.28,7.94 v38.43,7.94
VUSB
  Top 0.6: C17.1 14.98,43.16 USBMOD.5V
  Bottom 0.6: C9.1 arc90 9.84,41.69 9.84,43.1
  Bottom 1: JP1.3 4.76,41.75 6.11,43.1 9.84,43.1 USBMOD.5V

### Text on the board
Bottom: PCB by / WestfW
tPlace: 13 | 12 | 11 | 10 | 9 | 8 | 7 | 6 | 5 | 4 | 3 | 2 | 1 | 0
History: 20190605 by WestfW: Tag at "Version 0.1" | 20190603 by WestfW: dual footprints for reset switch. Connect Vin. | 20190602 by WestfW: Add fiducuals. Tweak silkscreen, backside cap packages. | 20190523 by WestfW: remove Aref, add backside bypass caps, simplify RESET | 20190520 by WestfW: Sort-of initial design, culled from UnoWifi2
To-Do: Prettify Silkscreen
_tSilk: L | SCL | R3 | SDA | PB3 | 13 | 12 | 11 | 10 | 9 | 8 | 7 | 6 | 5 | 4 | 3 | 2 | 1 | 0 | Digital | ON | C17 | PA7 | PA6 | Freeduino 4809 | C16 | R1 | USBMOD | RSTJ | USB3V | 20p | IN+ | IN- | SPI1 | C13 | 100n | PSel | VREG-3V3 | USB | 4u7 | OUT- | PA4 | PF3 | C14 | 32kHz | IN- | PA5 | PF2 | UPDI | 10k | R4 | VREG-5V | C12 | 100k | R2 | IN+ | - | OUT+ | OUT+ | OUT- | U1 | 100n | C3 | C7 | PC3 | RST | C11 | D1 | ATMEGA4809 | + | + | C2 | + | + | C1 | POWER | ANALOG | 6 | GND | 0 | AREF | PWR
_bplace: GND | 5V | TXD | RXD | DTR | 3V3 | Vusb | Copyright 2019 / by Bill Westfield | +5V | V5reg | UPDI | http://hackaday.io/project/165661 | Vdd Core | Vin | V3.3reg | Vdd Core

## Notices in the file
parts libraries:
Arduino-connectors: Copyright (c) 2016-2017 Arduino LLC. All right reserved.
